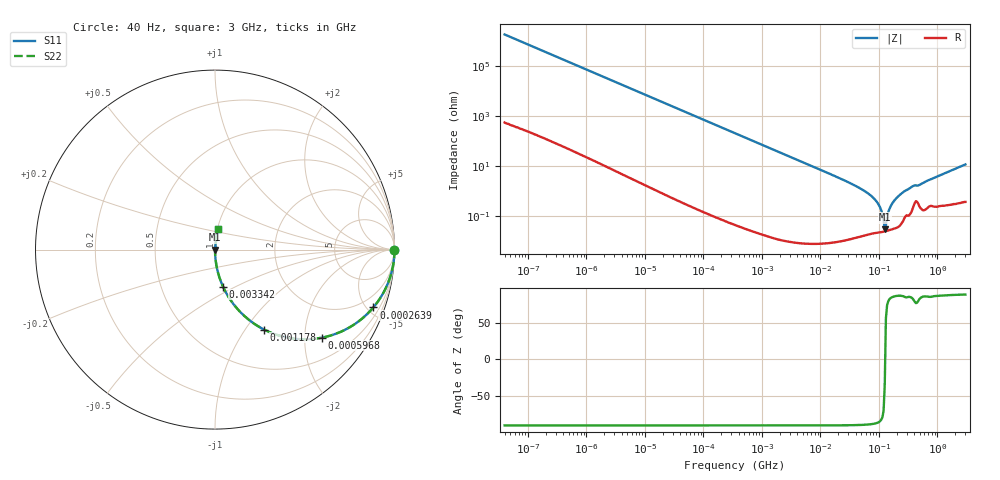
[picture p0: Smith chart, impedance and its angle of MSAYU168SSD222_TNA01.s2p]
! MSAYU168SSD222_TNA01  S-PARAMETER MODEL  ( General Type )
! Model Generated by TAIYO YUDEN Corporation (http://www.ty-top.com)
! Version 2.0
! TAIYO YUDEN Control No. 030711
! Copyright(c) 2003 TAIYO YUDEN CO.,LTD. All Rights Reserved.
! Product Description (link to TY-COMPAS)
! https://ds.yuden.co.jp/TYCOMPAS/or/detail?pn=MSAYU168SSD222KTNA01&u=M
! Products Name : Multilayer Ceramic Capacitors
! Characteristics :
!  Capacitance : 2200 pF , Rated Voltage : 50V
!  Case Size : 1.6 x 0.8 / 0.063 x 0.031 [mm/inch] , Thickness : 0.8 / 0.031 [mm/inch]
!  (Conditions: Temperature = 25 degC , DC Bias Current/Voltage = 0A / 0V)
! External Node Assignments :
!  1  o---| |---o  2
! GND o---------o GND
! Frequency Range : 40Hz  -  3GHz  [ 401 STEP ]
# MHz S RI R 50
! Freq[MHz].  S11 Real  S11 Imag  S21 Real  S21 Imag  S12 Real  S12 Imag  S22 Real  S22 Imag
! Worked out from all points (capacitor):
!   401 points, 40 Hz to 3 GHz, reference 50 ohm
!   read as one part in series: C = 2.2 nF near 44 Hz
!   lowest |Z| = 30.2 mohm at 125.6 MHz (marker M1)
!   series resonance near 127.4 MHz, so ESL is about 710 pH
!   S11 on the Smith chart (normalised r, x): 40 Hz: open; 263.9 kHz: 1.00, -5.48; 596.8 kHz: 1.00, -2.42; 1.178 MHz: 1.00, -1.23; 3.342 MHz: 1.00, -0.43; 3 GHz: 1.01, +0.23
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4e-05  1 -5.53e-05  2e-08 5.53e-05  2e-08 5.53e-05  1 -5.53e-05
7.9e-05  1 -0.000109  4.8e-08 0.000109  4.8e-08 0.000109  1 -0.000109
0.000834  1 -0.00115  1.7e-06 0.00115  1.7e-06 0.00115  1 -0.00115
0.017386  0.9994 -0.024  0.000583 0.024  0.000583 0.024  0.9994 -0.024
0.081206  0.9875 -0.1109  0.0125 0.1109  0.0125 0.1109  0.9875 -0.1109
0.263915  0.8824 -0.322  0.1176 0.322  0.1176 0.322  0.8824 -0.322
0.362475  0.7992 -0.4005  0.2008 0.4005  0.2008 0.4005  0.7992 -0.4005
0.596819  0.5948 -0.4908  0.4052 0.4908  0.4052 0.4908  0.5948 -0.4908
1.178032  0.2737 -0.4457  0.7263 0.4457  0.7263 0.4457  0.2737 -0.4457
3.341745  0.0448 -0.2066  0.9552 0.2066  0.9552 0.2066  0.0448 -0.2066
7.222098  0.00994 -0.0988  0.9901 0.0988  0.9901 0.0988  0.00994 -0.0988
32.2371  0.00056 -0.021  0.9994 0.021  0.9994 0.021  0.00056 -0.021
66.58224  0.000251 -0.00786  0.9997 0.00786  0.9997 0.00786  0.000251 -0.00786
95.68847  0.000232 -0.00327  0.9998 0.00327  0.9998 0.00327  0.000232 -0.00327
120.0322  0.000243 -0.000655  0.9998 0.000655  0.9998 0.000655  0.000243 -0.000655
125.5988  0.000249 -0.00017  0.9998 0.00017  0.9998 0.00017  0.000249 -0.00017
137.5184  0.000264 0.00088  0.9997 -0.00088  0.9997 -0.00088  0.000264 0.00088
150.5692  0.000283 0.00192  0.9997 -0.00192  0.9997 -0.00192  0.000283 0.00192
172.504  0.00032 0.00352  0.9997 -0.00352  0.9997 -0.00352  0.00032 0.00352
206.7996  0.000392 0.00579  0.9996 -0.00579  0.9996 -0.00579  0.000392 0.00579
356.2883  0.00165 0.0144  0.9984 -0.0144  0.9984 -0.0144  0.00165 0.0144
3000  0.0171 0.1147  0.9829 -0.1147  0.9829 -0.1147  0.0171 0.1147
